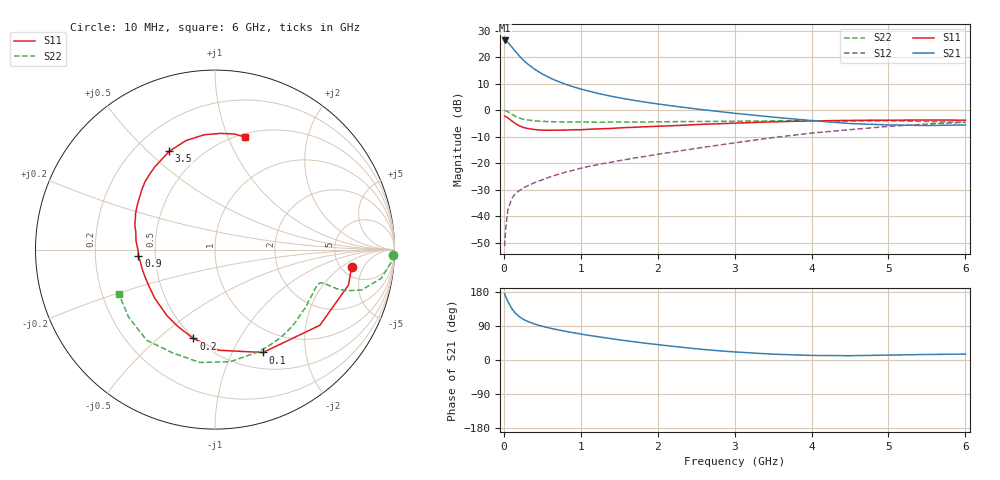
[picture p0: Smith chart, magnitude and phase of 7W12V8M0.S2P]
! Infineon Technologies  Discrete & RF Semiconductors
! BFS17W
! Si NPN RF Bipolar Junction Transistor in SOT323
! VCE = 12 V  IC = 8 mA
! Common Emitter S-Parameters:  August  1999
# GHz  S  MA  R  50
!  f  S11  S21  S12  S22
! GHz  MAG  ANG  MAG  ANG  MAG  ANG  MAG  ANG
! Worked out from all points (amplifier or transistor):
!   36 points, 10 MHz to 6 GHz, reference 50 ohm
!   highest |S21| = 26.4 dB at 10 MHz (marker M1)
!   |S21| within 3 dB of that: start of sweep to 118.6 MHz
!   unconditionally stable (mu >= 1): 488.2 MHz to 2.137 GHz; 5.62 GHz to end of sweep
!   at 250 MHz: K = 0.70, MSG = 24.2 dB, |S12| = -29.4 dB
!   at 1.4 GHz: K = 1.16, MAG = 10.0 dB, |S12| = -19.6 dB
!   at 6 GHz: K = 1.03, MAG = -1.6 dB, |S12| = -4.5 dB
!   S11 on the Smith chart (normalised r, x): 10 MHz: 6.18, -2.94; 100 MHz: 0.69, -1.32; 200 MHz: 0.49, -0.66; 900 MHz: 0.40, -0.04; 3.5 GHz: 0.34, +0.58; 6 GHz: 0.53, +1.15
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0.01  0.7676 -7.3  20.81 174.8  0.0027 79.4  0.9916 -1.6
0.02  0.7693 -14.9  20.58 169.5  0.0049 87.3  0.9821 -4.3
0.05  0.7207 -35.8  19.21 155.3  0.0126 76.6  0.9403 -9.8
0.1  0.6324 -65.0  15.92 136.8  0.021 63.3  0.8471 -15.4
0.15  0.5612 -87.8  12.93 123.5  0.0267 57.3  0.7659 -17.4
0.2  0.5097 -103.7  10.67 114.6  0.0302 56.2  0.7138 -17.8
0.25  0.475 -116.2  8.943 107.9  0.0338 54.1  0.679 -17.6
0.3  0.4549 -126.1  7.682 102.7  0.0368 55.1  0.6575 -17.4
0.4  0.4314 -141.1  5.954 94.8  0.0429 57.1  0.63 -17.2
0.5  0.4202 -151.3  4.844 88.9  0.0485 59.8  0.6167 -17.5
0.6  0.4185 -158.9  4.07 84.0  0.055 61.2  0.6085 -18.2
0.7  0.4198 -165.1  3.528 79.7  0.061 63.4  0.6035 -19.3
0.9  0.4279 -175.1  2.777 72.1  0.0732 65.3  0.5974 -22.0
1.1  0.4358 176.7  2.301 65.1  0.0866 67.0  0.5966 -25.3
1.3  0.448 169.7  1.966 59.1  0.0989 68.4  0.595 -29.1
1.6  0.4715 161.1  1.617 50.5  0.1178 70.1  0.5972 -35.0
2.2  0.5105 145.7  1.202 36.0  0.1627 73.2  0.6081 -48.6
2.8  0.5554 131.0  0.943 24.3  0.2198 73.6  0.6157 -63.6
3.5  0.604 115.0  0.741 15.4  0.3041 70.3  0.6302 -82.2
4.5  0.6426 95.4  0.56 11.4  0.4296 58.9  0.6221 -112.5
5.5  0.6533 80.6  0.514 14.6  0.5472 45.6  0.6108 -141.9
6  0.6487 75.0  0.527 15.6  0.5944 38.8  0.5903 -155.3
